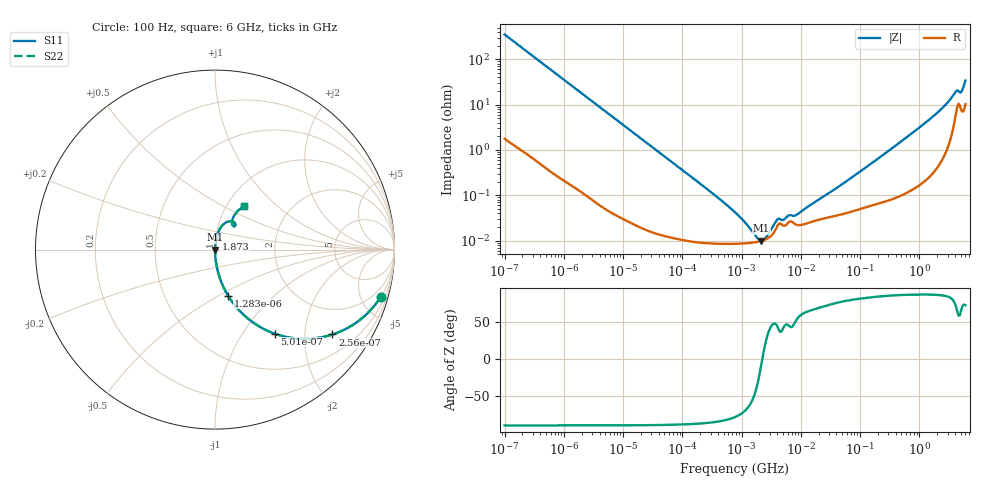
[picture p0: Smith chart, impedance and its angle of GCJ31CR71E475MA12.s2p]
!Murata Part Number: GCJ31CR71E475MA12
!These Parameters are Measured in Series Mode Connection
!Data Generated on Mar 13, 2026
!  o--ll--o
!Port1  Port2
!  o------o
!Operation Temp=25[degC], DC Bias Voltage=0[V]
!Freq. Start=100[Hz] Stop=6[GHz] 401[Steps]
# Hz S RI R 50
!Freq.(Hz) S11(Real) S11(Imag) S21(Real) S21(Imag) S12(Real) S12(Imag) S22(Real) S22(Imag)
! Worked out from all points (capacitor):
!   401 points, 100 Hz to 6 GHz, reference 50 ohm
!   read as one part in series: C = 4.52 uF near 109 Hz
!   lowest |Z| = 9.9 mohm at 2.169 MHz (marker M1)
!   series resonance near 2.239 MHz, so ESL is about 1.1 nH
!   S11 on the Smith chart (normalised r, x): 100 Hz: 1.04, -7.03; 256 Hz: 1.02, -2.75; 501 Hz: 1.01, -1.41; 1.283 kHz: 1.00, -0.55; 1.873 GHz: 1.01, +0.12; 6 GHz: 1.20, +0.65
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100  0.9241 -0.2624  0.0759 0.2624  0.0759 0.2624  0.9241 -0.2624
164  0.8211 -0.3807  0.1789 0.3807  0.1789 0.3807  0.8211 -0.3807
256  0.654 -0.473  0.346 0.473  0.346 0.473  0.654 -0.473
501  0.3331 -0.4686  0.6669 0.4686  0.6669 0.4686  0.3331 -0.4686
784  0.1707 -0.3734  0.8293 0.3734  0.8293 0.3734  0.1707 -0.3734
1283  0.0723 -0.2559  0.9277 0.2559  0.9277 0.2559  0.0723 -0.2559
2008  0.0314 -0.1712  0.9686 0.1712  0.9686 0.1712  0.0314 -0.1712
6433  0.00347 -0.0553  0.9965 0.0553  0.9965 0.0553  0.00347 -0.0553
40335  0.000215 -0.00891  0.9998 0.00891  0.9998 0.00891  0.000215 -0.00891
774597  8.49e-05 -0.000413  0.9999 0.000413  0.9999 0.000413  8.49e-05 -0.000413
1159002  8.68e-05 -0.000231  0.9999 0.000231  0.9999 0.000231  8.68e-05 -0.000231
1813585  9.31e-05 -7.02e-05  0.9999 7.02e-05  0.9999 7.02e-05  9.31e-05 -7.02e-05
2169299  9.84e-05 -1.06e-05  0.9999 1.06e-05  0.9999 1.06e-05  9.84e-05 -1.06e-05
2594782  0.000107 5.03e-05  0.9999 -5.03e-05  0.9999 -5.03e-05  0.000107 5.03e-05
4060267  0.000215 0.000202  0.9998 -0.000202  0.9998 -0.000202  0.000215 0.000202
8311524  0.000225 0.000286  0.9998 -0.000286  0.9998 -0.000286  0.000225 0.000286
1.555665e7  0.000261 0.000591  0.9997 -0.000591  0.9997 -0.000591  0.000261 0.000591
3.124326e8  0.000869 0.00977  0.9991 -0.00977  0.9991 -0.00977  0.000869 0.00977
1.873145e9  0.00717 0.06  0.9928 -0.06  0.9928 -0.06  0.00717 0.06
4.009986e9  0.0729 0.1567  0.9271 -0.1567  0.9271 -0.1567  0.0729 0.1567
5.016141e9  0.0959 0.1383  0.9041 -0.1383  0.9041 -0.1383  0.0959 0.1383
6e9  0.1643 0.2453  0.8357 -0.2453  0.8357 -0.2453  0.1643 0.2453
